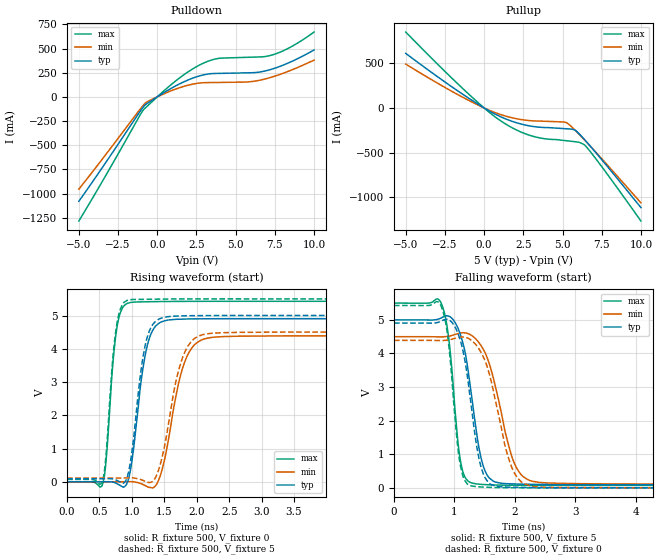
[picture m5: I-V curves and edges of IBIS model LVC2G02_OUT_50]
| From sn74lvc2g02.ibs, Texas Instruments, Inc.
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[Model]   LVC2G02_OUT_50
Model_type  Output
Vref =   0
Rref =   500
Cref =   50p
Vmeas =   2.5
| variable   typ   min   max
C_comp   8.06pF   6.00pF   11.21pF
| C_pullup   7.90pF   6.05pF   8.97pF
| C_pulldown   8.22pF   6.00pF   11.21pF
[Temperature Range]   40   100   -40
| Ambient temperature   25   85   -40
[Voltage range]   5   4.5   5.5
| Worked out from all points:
|   slope of the pulldown table from 0 to 0.75 V, typ, clamps not added: 9.96 ohm
|   slope of the pullup table from 0 to 0.75 V, typ, clamps not added: 10.3 ohm
|   rising waveform, R_fixture 500, V_fixture 0: 20-80 % time 193ps typ, 271ps min, 128ps max; typ from 0 V to 4.9 V
|   falling waveform, R_fixture 500, V_fixture 5: 20-80 % time 240ps typ, 350ps min, 163ps max; typ from 5 V to 0.093 V
|   rising waveform, R_fixture 500, V_fixture 5: 20-80 % time 185ps typ, 267ps min, 128ps max; typ from 0.093 V to 5 V
|   falling waveform, R_fixture 500, V_fixture 0: 20-80 % time 235ps typ, 339ps min, 164ps max; typ from 4.91 V to 0 V
[Pulldown]
| LVC2G02_OUT_50
|   Voltage   I(typ)   I(min)   I(max)
-5V       -1.081A    -955.5mA   -1.285A
-3.39V    -704.7mA   -619.9mA   -843.7mA
-930mV    -112.8mA   -94.73mA   -144.9mA
-620mV    -65.83mA   -48.59mA   -93.56mA
1.085V    105.9mA    75.6mA     153.4mA
2.27V     194.6mA    132.3mA    290.4mA
3.305V    238mA      148.1mA    373.1mA
4.035V    243.4mA    149.7mA    400.7mA
5.835V    249.3mA    155.6mA    410.1mA
7.275V    285.3mA    203.4mA    431.4mA
8.505V    361.5mA    274.3mA    515.5mA
10V       485.6mA    380.4mA    671.3mA
[Pullup]
| LVC2G02_OUT_50
|   Voltage   I(typ)   I(min)   I(max)
-5V       610.5mA    490.7mA    849.3mA
-1.235V   138.2mA    107.8mA    196.2mA
160mV     -16.77mA   -12.81mA   -24.19mA
1.06V     -98.65mA   -73.91mA   -144.2mA
2.035V    -163.6mA   -119.3mA   -243.7mA
3.01V     -203.9mA   -143mA     -311.3mA
3.855V    -218.8mA   -148.7mA   -344mA
5.275V    -233mA     -166.8mA   -367.2mA
5.82V     -250.4mA   -251.6mA   -378mA
6.475V    -367.7mA   -371.4mA   -425.5mA
7.705V    -621.4mA   -607.8mA   -704.7mA
10V       -1.115A    -1.061A    -1.264A
[Ramp]
| LVC2G02_OUT_50
| variable   typ   min   max
dV/dt_r   3.04/2.03E-10   2.74/2.85E-10   3.35/1.32E-10
dV/dt_f   3.02/2.54E-10   2.70/3.74E-10   3.33/1.75E-10
R_load = 500
[Rising Waveform]
| LVC2G02_OUT_50
R_fixture =   500
C_fixture =   0
L_fixture =   0
V_fixture =   0
V_fixture_min = 0
V_fixture_max = 0
|   Time   V(typ)   V(min)   V(max)
0s        -20.54nV   604.8nV    -4.292uV
545ps     372.2uV    -48.16uV   -89mV
770ps     -55.79mV   -291.2uV   4.651V
1ns       631.8mV    4.595mV    5.398V
1.245ns   4.156V     -154.9mV   5.414V
1.41ns    4.756V     40.74mV    5.419V
1.575ns   4.868V     1.399V     5.422V
1.85ns    4.895V     3.776V     5.425V
2.275ns   4.903V     4.351V     5.427V
24.99ns   4.904V     4.386V     5.427V
[Falling Waveform]
| LVC2G02_OUT_50
R_fixture =   500
C_fixture =   0
L_fixture =   0
V_fixture =   5
V_fixture_min = 4.5
V_fixture_max = 5.5
|   Time   V(typ)   V(min)   V(max)
0s        5V         4.5V       5.5V
785ps     5.061V     4.496V     5.485V
910ps     5.11V      4.515V     4.393V
1.055ns   4.768V     4.589V     1.418V
1.115ns   4.476V     4.614V     662.8mV
1.375ns   1.539V     4.391V     115.3mV
1.565ns   317.9mV    3.759V     91.01mV
1.995ns   115.4mV    718.1mV    75.16mV
2.4ns     100.7mV    160.7mV    72.11mV
24.99ns   92.94mV    113.9mV    72.02mV
[Rising Waveform]
| LVC2G02_OUT_50
R_fixture =   500
C_fixture =   0
L_fixture =   0
V_fixture =   5
V_fixture_min = 4.5
V_fixture_max = 5.5
|   Time   V(typ)   V(min)   V(max)
0s        92.92mV    113.9mV    72mV
540ps     93.26mV    113.8mV    -17.53mV
760ps     50.47mV    113.6mV    4.657V
955ps     359.9mV    117.7mV    5.473V
1.225ns   4.27V      -893.4uV   5.487V
1.395ns   4.863V     267.2mV    5.492V
1.565ns   4.967V     1.755V     5.496V
1.83ns    4.992V     3.963V     5.499V
2.255ns   4.999V     4.47V      5.5V
24.99ns   5V         4.5V       5.5V
[Falling Waveform]
| LVC2G02_OUT_50
R_fixture =   500
C_fixture =   0
L_fixture =   0
V_fixture =   0
V_fixture_min = 0
V_fixture_max = 0
|   Time   V(typ)   V(min)   V(max)
0s        4.907V     4.391V     5.429V
780ps     4.962V     4.387V     5.412V
895ps     5.011V     4.402V     4.425V
1.1ns     4.385V     4.488V     660mV
1.2ns     3.501V     4.472V     144.7mV
1.35ns    1.461V     4.272V     38.5mV
1.55ns    189.7mV    3.562V     16.75mV
1.95ns    18.88mV    605.8mV    3.346mV
2.315ns   7.42mV     36mV       379.9uV
24.99ns   11.78uV    17.27uV    9.473uV
